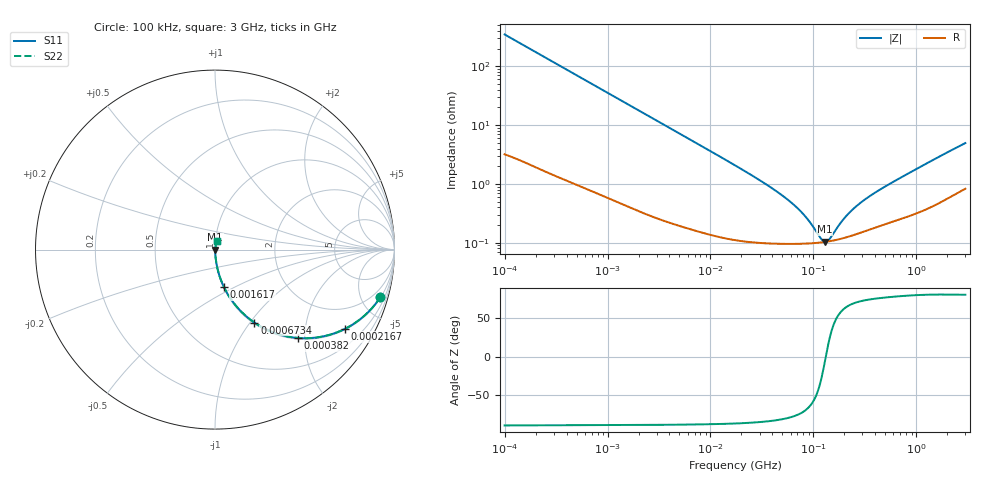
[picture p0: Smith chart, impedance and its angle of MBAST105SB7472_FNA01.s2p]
! MBAST105SB7472_FNA01  S-PARAMETER MODEL  ( Standard Model )
! Model Generated by TAIYO YUDEN Corporation (http://www.ty-top.com)
! Version 1.0
! TAIYO YUDEN Control No. 220601
! Copyright(c) 2013 TAIYO YUDEN CO.,LTD. All Rights Reserved.
! Product Description (link to TY-COMPAS)
! https://ds.yuden.co.jp/TYCOMPAS/or/detail?pn=MBAST105SB7472KFNA01&u=M
! Products Name : Multilayer Ceramic Capacitors
! Characteristics :
!  Capacitance : 4700 [pF] , Rated Voltage : 25 [V] , TCC : X7R
!  Case Size : 1.0 x 0.5 / 0.039 x 0.02 [mm/inch] , Thickness : 0.5 / 0.02 [mm/inch]
!  (Conditions: Temperature = 25 [degC] , DC Bias Voltage = 0 [V])
! External Node Assignments :
!  1  o---| |---o  2
! GND o---------o GND
! Frequency Range : 100kHz  -  3GHz  [ 401 STEP ]
# MHZ S RI R 50
! Freq[MHz].  S11 Real  S11 Imag  S21 Real  S21 Imag  S12 Real  S12 Imag  S22 Real  S22 Imag
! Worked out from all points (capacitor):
!   401 points, 100 kHz to 3 GHz, reference 50 ohm
!   read as one part in series: C = 4.55 nF near 105.3 kHz
!   lowest |Z| = 104 mohm at 129.3 MHz (marker M1)
!   series resonance near 132.1 MHz, so ESL is about 320 pH
!   S11 on the Smith chart (normalised r, x): 100 kHz: 1.06, -6.98; 216.7 kHz: 1.04, -3.24; 382 kHz: 1.02, -1.84; 673.4 kHz: 1.02, -1.05; 1.617 MHz: 1.01, -0.44; 3 GHz: 1.02, +0.10
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0.1  0.922 -0.2636  0.078 0.2636  0.078 0.2636  0.922 -0.2636
0.147195  0.847 -0.3549  0.153 0.3549  0.153 0.3549  0.847 -0.3549
0.216663  0.7216 -0.4427  0.2784 0.4427  0.2784 0.4427  0.7216 -0.4427
0.381967  0.4599 -0.4921  0.5401 0.4921  0.5401 0.4921  0.4599 -0.4921
0.562235  0.2857 -0.4448  0.7143 0.4448  0.7143 0.4448  0.2857 -0.4448
0.673391  0.2197 -0.4067  0.7803 0.4067  0.7803 0.4067  0.2197 -0.4067
1.017073  0.1126 -0.3081  0.8874 0.3081  0.8874 0.3081  0.1126 -0.3081
1.61742  0.0498 -0.2087  0.9502 0.2087  0.9502 0.2087  0.0498 -0.2087
3.161081  0.0151 -0.1115  0.9849 0.1115  0.9849 0.1115  0.0151 -0.1115
17.7727  0.0015 -0.0201  0.9985 0.0201  0.9985 0.0201  0.0015 -0.0201
34.73492  0.00107 -0.00979  0.9989 0.00979  0.9989 0.00979  0.00107 -0.00979
53.83243  0.000985 -0.00566  0.999 0.00566  0.999 0.00566  0.000985 -0.00566
75.25761  0.000968 -0.00328  0.999 0.00328  0.999 0.00328  0.000968 -0.00328
97.38194  0.000981 -0.00171  0.999 0.00171  0.999 0.00171  0.000981 -0.00171
116.6348  0.00101 -0.000689  0.999 0.000689  0.999 0.000689  0.00101 -0.000689
129.3002  0.00103 -0.000118  0.999 0.000118  0.999 0.000118  0.00103 -0.000118
143.341  0.00106 0.000449  0.9989 -0.000449  0.9989 -0.000449  0.00106 0.000449
195.2919  0.0012 0.00218  0.9988 -0.00218  0.9988 -0.00218  0.0012 0.00218
252.704  0.00138 0.00371  0.9986 -0.00371  0.9986 -0.00371  0.00138 0.00371
353.2796  0.00171 0.00596  0.9983 -0.00596  0.9983 -0.00596  0.00171 0.00596
547.5153  0.00227 0.00967  0.9977 -0.00967  0.9977 -0.00967  0.00227 0.00967
3000  0.0106 0.048  0.9894 -0.048  0.9894 -0.048  0.0106 0.048
